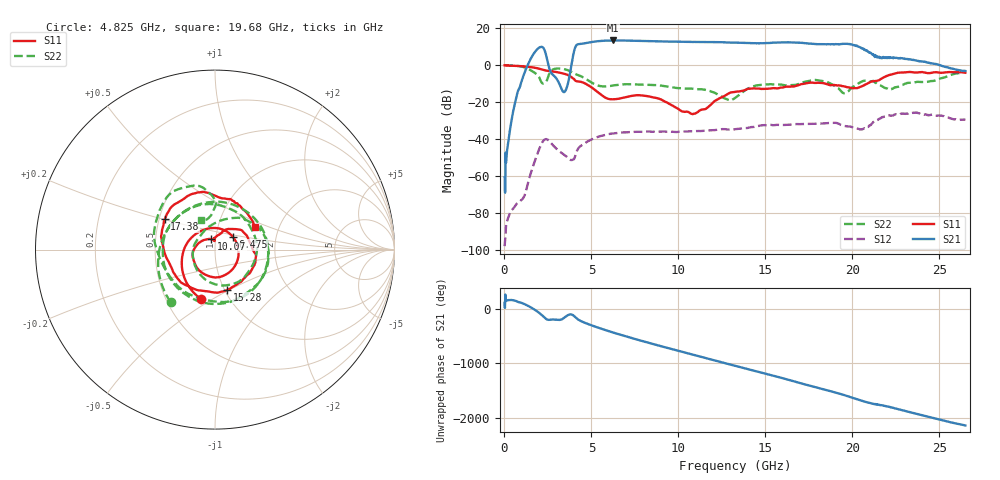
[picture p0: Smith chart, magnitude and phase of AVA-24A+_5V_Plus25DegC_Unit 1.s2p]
!Mini-Circuits Laboratory
!Date: 7/17/2015 at 11:12:29 AM
!S2P DATA File Format
!Type: MMIC Amplifier
!Model: AVA-24A+
!S/N: Unit 1
!Fixture: Unit soldered on TB-547+ D/C 1421, no port extension
!PIN OUT: PORT 1 - PIN 2, PORT 2 - PIN 5, GROUND - PADDLE, DC POWER SUPPLY - PINS 7,8, NOT CONNECTED - PINS 1,3,4,6
!TEST CONDITIONS: Temp= 25 (Deg C) RF Power= -25.00 (dBm) V limit=5(V) I limit=250(mA) Z=50 OHM
!WAFER/LOT#: CP164 DATE CODE: N/A
!Network Analyzer: PNA-X N5242A S/N 71404 CAL DUE: 12/5/2015
!P.Supply/Multimeter: HP E3632A S/N 63249 CAL DUE: 12/11/2015
!Power Meter: Agilent U2000A S/N 74434 CAL DUE: 10/17/2015
# Hz  S  dB  R  50
!Frequency  S11 dB  S11 Deg  S21 dB  S21 Deg  S12 dB  S12 Deg  S22 dB  S22 Deg
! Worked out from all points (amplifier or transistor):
!   988 points, 10 MHz to 26.5 GHz, reference 50 ohm
!   highest |S21| = 13.4 dB at 6.225 GHz (marker M1)
!   |S21| within 3 dB of that: 4.106 GHz to 20.23 GHz (16.13 GHz wide, 133 % of centre)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
!   unconditionally stable (mu >= 1): start of sweep to end of sweep
!   at 5.925 GHz: K = 7.28, MAG = 13.7 dB, |S12| = -37.4 dB
!   at 14.18 GHz: K = 5.39, MAG = 12.4 dB, |S12| = -33.5 dB
!   at 26.5 GHz: K = 7.67, MAG = 1.3 dB, |S12| = -29.5 dB
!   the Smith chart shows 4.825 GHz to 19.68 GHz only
!   S11 on the Smith chart (normalised r, x): 4.825 GHz: 0.74, -0.45; 6.475 GHz: 1.21, +0.17; 10.07 GHz: 0.95, +0.11; 15.28 GHz: 1.03, -0.49; 17.38 GHz: 0.54, +0.20; 19.68 GHz: 1.50, +0.41
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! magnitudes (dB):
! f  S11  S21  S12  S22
! 10 MHz  0.0  -60.6  -97.9  0.0
! 100 MHz  -0.2  -52.2  -86.0  0.0
! 600 MHz  -0.3  -20.8  -76.3  -0.2
! 1.55 GHz  -1.1  4.2  -57.4  -2.9
! 2.35 GHz  -2.8  7.0  -40.0  -9.4
! 3.45 GHz  -4.7  -14.5  -48.6  -2.2
! 4.1 GHz  -8.5  10.3  -48.1  -4.8
! 4.425 GHz  -9.0  11.6  -43.4  -6.1
! 4.825 GHz  -10.9  12.2  -41.0  -8.3
! 6.225 GHz  -18.4  13.4  -36.9  -11.0
! 6.475 GHz  -18.2  13.4  -36.6  -10.7
! 8.85 GHz  -18.0  12.9  -35.8  -10.8
! 10.07 GHz  -24.2  12.7  -35.9  -12.4
! 10.93 GHz  -26.2  12.6  -35.7  -12.8
! 13.28 GHz  -14.4  12.2  -34.6  -17.6
! 15.28 GHz  -12.6  12.1  -32.3  -10.3
! 17.38 GHz  -9.7  11.9  -31.8  -8.8
! 17.68 GHz  -9.4  11.6  -31.7  -8.1
! 19.68 GHz  -11.9  11.6  -33.0  -14.8
! 20.73 GHz  -10.5  8.4  -34.2  -8.3
! 22.1 GHz  -5.4  4.2  -27.1  -13.0
! 26.5 GHz  -4.1  -3.1  -29.5  -3.8
